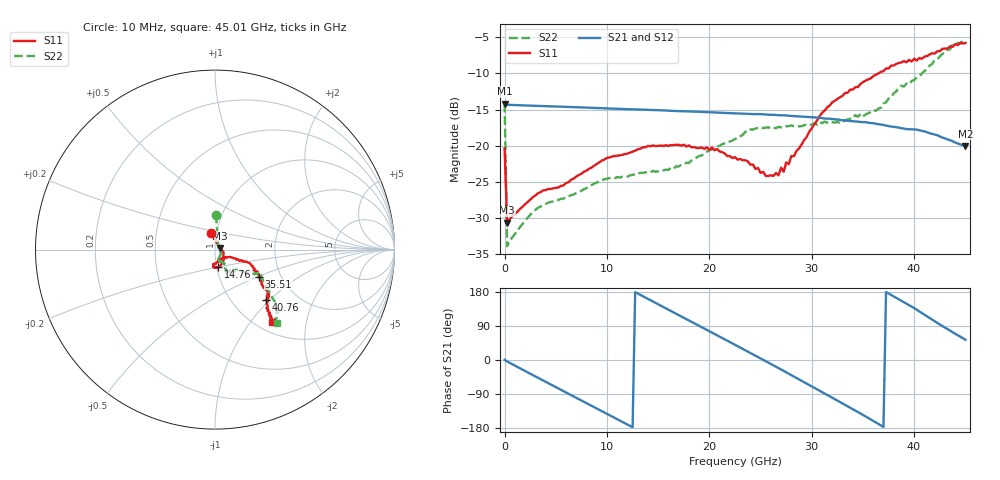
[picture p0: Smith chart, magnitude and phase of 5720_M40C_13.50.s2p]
! Device:  ADRF5720
! Description: 0.5dB LSB GaAs MMIC 6-bit Digital Attenuator
! Frequency:  0.000009 -  40 GHz
! Ports:
!	RF1	= Port 1
!	RF2	= Port 2
! Vdd:  3.3 Volt
! Vss:  -3.3 Volt
! Control:  0/3.3 Volt
! State:  13.50 dB attenuation
! Data:  The device was measured using G-S-G Probes on a matrix board.
!  Data was collected using an calibrated 4 port network analyzer.
!  The reference plane for this measurement is at the launchers.
! Note:  Analog Devices supplies this data as a sample of measured data
!  for this product.  Your particular data for this product may vary.
!  Data was taken at -40 degrees C.
!  Analog Devices reserves the right to change this data at anytime.
# GHZ S DB R 45.0
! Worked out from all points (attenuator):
!   181 points, 10 MHz to 45.01 GHz, reference 45 ohm
!   highest |S21| = -14.16 dB at 10 MHz (marker M1); lowest = -20.0 dB at 45.01 GHz (marker M2)
!   lowest |S11| = -30.6 dB at 260 MHz (marker M3), VSWR 1.06, Z = 47.6 + j0.821 ohm
!   |S11| at or under -10 dB: start of sweep to 36.52 GHz
!   |S22| runs from -33.9 to -5.4 dB; largest |S21 - S12| = 0.00074
!   S11 on the Smith chart (normalised r, x): 10 MHz: 0.94, +0.18; 14.76 GHz: 1.02, -0.20; 35.51 GHz: 1.55, -0.51; 40.76 GHz: 1.42, -0.95; 45.01 GHz: 1.16, -1.28
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0.01  -20.37 104.7  -14.16 0.3  -14.18 0.2  -14.19 88.3
0.26  -30.64 17.1  -14.34 -3.9  -14.36 -3.9  -33.87 22.4
3.26  -26.56 -13.4  -14.49 -46.8  -14.52 -46.9  -28.57 -30.4
5.76  -25.48 -29.8  -14.61 -82.2  -14.63 -82.2  -27.30 -50.0
7.76  -23.58 -44.0  -14.71 -110.4  -14.73 -110.5  -26.00 -64.3
11.26  -21.32 -61.5  -14.90 -159.8  -14.92 -159.9  -24.38 -73.5
14.76  -20.03 -79.1  -15.08 150.6  -15.10 150.5  -23.59 -72.4
15.26  -19.97 -81.2  -15.10 143.5  -15.12 143.4  -23.49 -71.6
19.01  -20.33 -93.3  -15.31 90.2  -15.33 90.1  -21.42 -59.5
20.26  -20.24 -94.7  -15.38 72.3  -15.40 72.2  -20.49 -57.6
22.76  -21.92 -95.8  -15.53 36.5  -15.56 36.4  -18.93 -60.3
23.76  -22.15 -89.3  -15.60 22.2  -15.62 22.1  -18.06 -61.5
25.51  -24.16 -64.4  -15.68 -3.3  -15.70 -3.4  -17.50 -61.7
26.76  -24.08 -45.5  -15.78 -21.5  -15.80 -21.7  -17.39 -62.3
27.01  -23.02 -42.7  -15.79 -25.1  -15.82 -25.2  -17.45 -64.0
30.26  -17.02 -22.5  -16.08 -73.4  -16.10 -73.5  -16.86 -62.4
32.01  -13.99 -21.7  -16.31 -99.6  -16.34 -99.8  -16.74 -56.3
35.51  -10.84 -31.5  -16.81 -152.9  -16.83 -153.1  -15.50 -42.1
37.76  -8.93 -38.3  -17.34 171.8  -17.37 171.6  -13.30 -36.8
40.76  -7.98 -44.7  -17.94 123.8  -17.97 123.6  -10.01 -32.0
43.76  -6.33 -49.8  -19.36 73.3  -19.39 73.1  -6.07 -44.8
45.01  -5.79 -52.1  -20.01 53.6  -20.04 53.4  -5.45 -50.0
